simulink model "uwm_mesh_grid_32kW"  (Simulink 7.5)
settings: Solver=ode45  StartTime=0.0  StopTime=6.0  RelTol=1e-4
undefined symbols (not defined in the file or in its folder): bits, D1, Delta
libraries: powerlib x76, powerlib_extras x11, dspswit3 x4
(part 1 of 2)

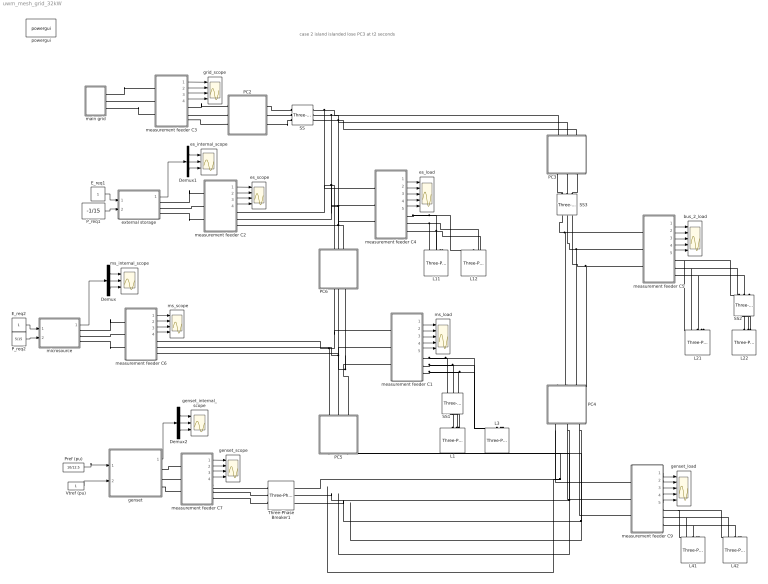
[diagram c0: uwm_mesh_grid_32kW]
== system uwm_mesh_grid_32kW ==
  note: case 2 island islanded lose PC3 at t2 seconds
  " es_scope" : Scope  NumInputPorts=4
  " ms_scope" : Scope  NumInputPorts=4
  Demux : Demux  Outputs=3
  Demux1 : Demux  Outputs=3
  Demux2 : Demux  Outputs=3
  E_req1 : Constant  OutDataType=fixdt(1, 16)  OutScaling=2^0
  E_req2 : Constant  OutDataType=fixdt(1, 16)  OutScaling=2^0
  L{1,3,11..12,21..22,41..42} (8 alike) : powerlib/Elements/Three-Phase Series RLC Load  DialogController=POWERSYS.PowerSysDialog  PhysicalDomain=powersysdomain  SubClassName=unknown  LeftPortType=p1  RightPortType=p1  LConnTagsString=A|B|C  Configuration=Y (grounded)  NominalVoltage=208  NominalFrequency=60  ActivePower=4000  InductivePower=0  CapacitivePower=0  Measurements=None
  PC2 : Subsystem  mask{R=.002810, L=.000679, C=2894.3}
  PC3 : Subsystem  mask{R=0.027352, L=.006600, C=288.6}
  PC4 : Subsystem  mask{R=.01688, L=.004070, C=336.7}
  PC5 : Subsystem  mask{R=.002600, L=.000640, C=2020.1}
  PC6 : Subsystem  mask{R=.013700, L=.003300, C=577.2}
  P_req1 : Constant  Value=-1/15  OutDataType=fixdt(1, 16)  OutScaling=2^0
  P_req2 : Constant  Value=5/15  OutDataType=fixdt(1, 16)  OutScaling=2^0
  Pref (pu) : Constant  Value=10/12.5  OutDataType=sfix(16)  OutScaling=2^0
  SS : powerlib/Elements/Three-Phase Breaker  DialogController=POWERSYS.PowerSysDialog  SystemSampleTime=-1  InitialState=closed  SwitchA=on  SwitchB=on  SwitchC=on  SwitchTimes=[3]  External=off  BreakerResistance=.001  SnubberResistance=1e6  SnubberCapacitance=inf  Measurements=None
  SS1 : powerlib/Elements/Three-Phase Breaker  DialogController=POWERSYS.PowerSysDialog  SystemSampleTime=-1  InitialState=closed  SwitchA=on  SwitchB=on  SwitchC=on  SwitchTimes=[50]  External=off  BreakerResistance=.001  SnubberResistance=1e6  SnubberCapacitance=inf  Measurements=None
  SS2 : powerlib/Elements/Three-Phase Breaker  DialogController=POWERSYS.PowerSysDialog  SystemSampleTime=-1  InitialState=closed  SwitchA=on  SwitchB=on  SwitchC=on  SwitchTimes=[50]  External=off  BreakerResistance=.00001  SnubberResistance=1e10  SnubberCapacitance=inf  Measurements=None
  SS3 : powerlib/Elements/Three-Phase Breaker  DialogController=POWERSYS.PowerSysDialog  SystemSampleTime=-1  InitialState=closed  SwitchA=on  SwitchB=on  SwitchC=on  SwitchTimes=[50]  External=off  BreakerResistance=.00001  SnubberResistance=1e10  SnubberCapacitance=inf  Measurements=None
  Three-Phase Breaker1 : powerlib/Elements/Three-Phase Breaker  DialogController=POWERSYS.PowerSysDialog  SystemSampleTime=-1  InitialState=closed  SwitchA=on  SwitchB=on  SwitchC=on  SwitchTimes=[50]  External=off  BreakerResistance=0.001  SnubberResistance=1e6  SnubberCapacitance=inf  Measurements=None
  Vtref (pu) : Constant  OutDataType=sfix(16)  OutScaling=2^0
  bus_2_load : Scope  NumInputPorts=5
  es_internal_scope : Scope  NumInputPorts=3
  es_load : Scope  NumInputPorts=5
  external storage : Subsystem  AncestorBlock=|
      | UWM_blocks/inverter-based
      | DG (simplified)
      | 208V - 15kVA
  genset : Subsystem
  genset_internal_scope : Scope  NumInputPorts=3
  genset_load : Scope  NumInputPorts=5
  genset_scope : Scope  NumInputPorts=4
  grid_scope : Scope  NumInputPorts=4
  main grid : Subsystem
  measurement feeder C1 : Subsystem
  measurement feeder C2 : Subsystem
  measurement feeder C3 : Subsystem
  measurement feeder C4 : Subsystem
  measurement feeder C5 : Subsystem
  measurement feeder C6 : Subsystem
  measurement feeder C7 : Subsystem
  measurement feeder C9 : Subsystem
  microsource : Subsystem  AncestorBlock=|
      | UWM_blocks/inverter-based
      | DG (simplified)
      | 208V - 15kVA
  ms_internal_scope : Scope  NumInputPorts=3
  ms_load : Scope  NumInputPorts=5
  powergui : powerlib/powergui  Priority=1  SystemSampleTime=-1  SimulationMode=Discrete  SampleTime=50e-6  frequency=60  SPID=off  DisableSnubberDevices=off  DisableRonSwitches=off  DisableVfSwitches=off  SwTol=0  Interpol=off  frequencyindice=60  echomessages=off  HookPort=off  DisplayEquations=off  FunctionMessages=off  EnableUseOfTLC=off  x0status=steady  RestoreLinks=no  ResistiveCurrentMeasurement=off  Frange=[0:2:500]  Ylog=off  Xlog=on  ShowGrid=off  save=off  variable=ZData  ZoomFFT=on  StartTime=0.0  cycles=1  DisplayStyle=1  fundamental=60  FreqAxis=off  MaxFrequency=1000  frequencyindicesteady=1  RmsSteady=2  display=off  Ts=0  methode=off
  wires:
  measurement feeder C3/1(Vabc) -> grid_scope/1
  measurement feeder C3/2(Iabc) -> grid_scope/2
  measurement feeder C3/3(PQ) -> grid_scope/3
  measurement feeder C3/4(RMS (V-I)) -> grid_scope/4
  measurement feeder C6/1(Vabc) -> " ms_scope"/1
  measurement feeder C6/2(Iabc) -> " ms_scope"/2
  measurement feeder C6/3(PQ) -> " ms_scope"/3
  measurement feeder C6/4(RMS (V-I)) -> " ms_scope"/4
  P_req2/1 -> microsource/2(P_req)
  E_req2/1 -> microsource/1(E_req)
  Demux/2 -> ms_internal_scope/2
  Demux/1 -> ms_internal_scope/1
  Demux/3 -> ms_internal_scope/3
  microsource/1(m) -> Demux/1
  P_req1/1 -> external storage/2(P_req)
  E_req1/1 -> external storage/1(E_req)
  Demux1/2 -> es_internal_scope/2
  Demux1/1 -> es_internal_scope/1
  Demux1/3 -> es_internal_scope/3
  external storage/1(m) -> Demux1/1
  measurement feeder C2/1(Vabc) -> " es_scope"/1
  measurement feeder C2/2(Iabc) -> " es_scope"/2
  measurement feeder C2/3(PQ) -> " es_scope"/3
  measurement feeder C2/4(RMS (V-I)) -> " es_scope"/4
  measurement feeder C4/5(w) -> es_load/5
  measurement feeder C4/4(RMS (V-I)) -> es_load/4
  measurement feeder C4/3(PQ) -> es_load/3
  measurement feeder C4/2(Iabc) -> es_load/2
  measurement feeder C4/1(Vabc) -> es_load/1
  measurement feeder C1/5(w) -> ms_load/5
  measurement feeder C1/4(RMS (V-I)) -> ms_load/4
  measurement feeder C1/3(PQ) -> ms_load/3
  measurement feeder C1/2(Iabc) -> ms_load/2
  measurement feeder C1/1(Vabc) -> ms_load/1
  measurement feeder C5/5(w) -> bus_2_load/5
  measurement feeder C5/4(RMS (V-I)) -> bus_2_load/4
  measurement feeder C5/3(PQ) -> bus_2_load/3
  measurement feeder C5/2(Iabc) -> bus_2_load/2
  measurement feeder C5/1(Vabc) -> bus_2_load/1
  measurement feeder C7/1(Vabc) -> genset_scope/1
  measurement feeder C7/2(Iabc) -> genset_scope/2
  measurement feeder C7/3(PQ) -> genset_scope/3
  measurement feeder C7/4(RMS (V-I)) -> genset_scope/4
  measurement feeder C9/5(w) -> genset_load/5
  measurement feeder C9/4(RMS (V-I)) -> genset_load/4
  measurement feeder C9/3(PQ) -> genset_load/3
  measurement feeder C9/1(Vabc) -> genset_load/1
  measurement feeder C9/2(Iabc) -> genset_load/2
  Vtref (pu)/1 -> genset/2(Ereq)
  Pref (pu)/1 -> genset/1(Preq)
  Demux2/2 -> genset_internal_scope/2
  Demux2/1 -> genset_internal_scope/1
  Demux2/3 -> genset_internal_scope/3
  genset/1(m) -> Demux2/1
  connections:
  SS/RConn3 -- measurement feeder C4/LConn3 -- measurement feeder C2/RConn3 -- PC6/RConn3 -- PC3/RConn3
  SS/RConn2 -- measurement feeder C4/LConn2 -- measurement feeder C2/RConn2 -- PC6/RConn2 -- PC3/RConn2
  SS/RConn1 -- measurement feeder C4/LConn1 -- measurement feeder C2/RConn1 -- PC6/RConn1 -- PC3/RConn1
  measurement feeder C4/RConn1 -- L12/LConn1 -- L11/LConn1
  measurement feeder C4/RConn2 -- L12/LConn2 -- L11/LConn2
  measurement feeder C4/RConn3 -- L12/LConn3 -- L11/LConn3
  measurement feeder C1/RConn1 -- L3/LConn1 -- SS1/LConn1
  measurement feeder C1/RConn2 -- L3/LConn2 -- SS1/LConn2
  measurement feeder C1/RConn3 -- L3/LConn3 -- SS1/LConn3
  measurement feeder C5/RConn1 -- SS2/LConn1 -- L21/LConn1
  measurement feeder C5/RConn2 -- SS2/LConn2 -- L21/LConn2
  measurement feeder C5/RConn3 -- SS2/LConn3 -- L21/LConn3
  measurement feeder C5/LConn1 -- PC4/RConn1 -- SS3/RConn1
  measurement feeder C5/LConn2 -- PC4/RConn2 -- SS3/RConn2
  measurement feeder C5/LConn3 -- PC4/RConn3 -- SS3/RConn3
  PC4/LConn1 -- measurement feeder C9/LConn1 -- Three-Phase Breaker1/RConn1 -- PC5/LConn1
  PC4/LConn2 -- measurement feeder C9/LConn2 -- Three-Phase Breaker1/RConn2 -- PC5/LConn2
  PC4/LConn3 -- measurement feeder C9/LConn3 -- Three-Phase Breaker1/RConn3 -- PC5/LConn3
  measurement feeder C9/RConn1 -- L41/LConn1 -- L42/LConn1
  measurement feeder C9/RConn2 -- L41/LConn2 -- L42/LConn2
  measurement feeder C9/RConn3 -- L41/LConn3 -- L42/LConn3
  PC5/RConn1 -- measurement feeder C6/RConn1 -- measurement feeder C1/LConn1 -- PC6/LConn1
  PC5/RConn2 -- measurement feeder C6/RConn2 -- measurement feeder C1/LConn2 -- PC6/LConn2
  microsource/RConn1 -- measurement feeder C6/LConn1
  PC5/RConn3 -- measurement feeder C6/RConn3 -- PC6/LConn3 -- measurement feeder C1/LConn3
  microsource/RConn2 -- measurement feeder C6/LConn2
  microsource/RConn3 -- measurement feeder C6/LConn3
  main grid/RConn2 -- measurement feeder C3/LConn2
  main grid/RConn1 -- measurement feeder C3/LConn1
  measurement feeder C3/LConn3 -- main grid/RConn3
  external storage/RConn2 -- measurement feeder C2/LConn2
  external storage/RConn1 -- measurement feeder C2/LConn1
  external storage/RConn3 -- measurement feeder C2/LConn3
  L1/LConn2 -- SS1/RConn2
  L1/LConn3 -- SS1/RConn3
  L1/LConn1 -- SS1/RConn1
  L22/LConn2 -- SS2/RConn2
  L22/LConn3 -- SS2/RConn3
  L22/LConn1 -- SS2/RConn1
  genset/RConn3 -- measurement feeder C7/LConn3
  genset/RConn1 -- measurement feeder C7/LConn1
  genset/RConn2 -- measurement feeder C7/LConn2
  measurement feeder C7/RConn1 -- Three-Phase Breaker1/LConn1
  Three-Phase Breaker1/LConn2 -- measurement feeder C7/RConn2
  Three-Phase Breaker1/LConn3 -- measurement feeder C7/RConn3
  measurement feeder C3/RConn1 -- PC2/LConn1
  measurement feeder C3/RConn2 -- PC2/LConn2
  measurement feeder C3/RConn3 -- PC2/LConn3
  PC2/RConn2 -- SS/LConn2
  PC2/RConn1 -- SS/LConn1
  SS/LConn3 -- PC2/RConn3
  SS3/LConn2 -- PC3/LConn2
  SS3/LConn3 -- PC3/LConn3
  SS3/LConn1 -- PC3/LConn1

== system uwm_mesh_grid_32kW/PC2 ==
  Ground : powerlib/Elements/Ground  DialogController=POWERSYS.PowerSysDialog  PhysicalDomain=powersysdomain  SubClassName=unknown  LeftPortType=p1  RightPortType=p1  LConnTagsString=a
  Three-Phase Parallel RLC Branch : powerlib/Elements/Three-Phase Parallel RLC Branch  DialogController=POWERSYS.PowerSysDialog  PhysicalDomain=powersysdomain  SubClassName=unknown  LeftPortType=p1  RightPortType=p1  LConnTagsString=A|B|C  RConnTagsString=A|B|C  BranchType=C  Resistance=1  Inductance=1e-3  Capacitance=1/(C*2*pi*60)  Measurements=None
  Three-Phase Series RLC Branch3 : powerlib/Elements/Three-Phase Series RLC Branch  DialogController=POWERSYS.PowerSysDialog  PhysicalDomain=powersysdomain  SubClassName=unknown  LeftPortType=p1  RightPortType=p1  LConnTagsString=A|B|C  RConnTagsString=A|B|C  BranchType=RL  Resistance=R  Inductance=L/(2*pi*60)  Capacitance=1/(336*2*pi*60)  Measurements=None
  A* : PMIOPort  Tag=PMCPort  Port=1  Side=Right
  B* : PMIOPort  Tag=PMCPort  Port=2  Side=Right
  C* : PMIOPort  Tag=PMCPort  Port=3  Side=Right
  A : PMIOPort  Tag=PMCPort  Port=4  Side=Left
  B : PMIOPort  Tag=PMCPort  Port=5  Side=Left
  C : PMIOPort  Tag=PMCPort  Port=6  Side=Left
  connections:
  Three-Phase Parallel RLC Branch/LConn1 -- A*/RConn1 -- Three-Phase Series RLC Branch3/LConn1
  Three-Phase Parallel RLC Branch/LConn2 -- B*/RConn1 -- Three-Phase Series RLC Branch3/LConn2
  Three-Phase Parallel RLC Branch/LConn3 -- C*/RConn1 -- Three-Phase Series RLC Branch3/LConn3
  Three-Phase Series RLC Branch3/RConn1 -- A/RConn1
  Three-Phase Series RLC Branch3/RConn2 -- B/RConn1
  Three-Phase Series RLC Branch3/RConn3 -- C/RConn1
  Ground/LConn1 -- Three-Phase Parallel RLC Branch/RConn2 -- Three-Phase Parallel RLC Branch/RConn3 -- Three-Phase Parallel RLC Branch/RConn1

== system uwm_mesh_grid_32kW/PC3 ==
  Ground : powerlib/Elements/Ground  DialogController=POWERSYS.PowerSysDialog  PhysicalDomain=powersysdomain  SubClassName=unknown  LeftPortType=p1  RightPortType=p1  LConnTagsString=a
  Three-Phase Parallel RLC Branch : powerlib/Elements/Three-Phase Parallel RLC Branch  DialogController=POWERSYS.PowerSysDialog  PhysicalDomain=powersysdomain  SubClassName=unknown  LeftPortType=p1  RightPortType=p1  LConnTagsString=A|B|C  RConnTagsString=A|B|C  BranchType=C  Resistance=1  Inductance=1e-3  Capacitance=1/(C*2*pi*60)  Measurements=None
  Three-Phase Series RLC Branch3 : powerlib/Elements/Three-Phase Series RLC Branch  DialogController=POWERSYS.PowerSysDialog  PhysicalDomain=powersysdomain  SubClassName=unknown  LeftPortType=p1  RightPortType=p1  LConnTagsString=A|B|C  RConnTagsString=A|B|C  BranchType=RL  Resistance=R  Inductance=L/(2*pi*60)  Capacitance=1/(336*2*pi*60)  Measurements=None
  A* : PMIOPort  Tag=PMCPort  Port=1  Side=Right
  B* : PMIOPort  Tag=PMCPort  Port=2  Side=Right
  C* : PMIOPort  Tag=PMCPort  Port=3  Side=Right
  A : PMIOPort  Tag=PMCPort  Port=4  Side=Left
  B : PMIOPort  Tag=PMCPort  Port=5  Side=Left
  C : PMIOPort  Tag=PMCPort  Port=6  Side=Left
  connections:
  Three-Phase Parallel RLC Branch/LConn1 -- A*/RConn1 -- Three-Phase Series RLC Branch3/LConn1
  Three-Phase Parallel RLC Branch/LConn2 -- B*/RConn1 -- Three-Phase Series RLC Branch3/LConn2
  Three-Phase Parallel RLC Branch/LConn3 -- C*/RConn1 -- Three-Phase Series RLC Branch3/LConn3
  Three-Phase Series RLC Branch3/RConn1 -- A/RConn1
  Three-Phase Series RLC Branch3/RConn2 -- B/RConn1
  Three-Phase Series RLC Branch3/RConn3 -- C/RConn1
  Ground/LConn1 -- Three-Phase Parallel RLC Branch/RConn2 -- Three-Phase Parallel RLC Branch/RConn1 -- Three-Phase Parallel RLC Branch/RConn3

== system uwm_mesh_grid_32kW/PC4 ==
  Ground : powerlib/Elements/Ground  DialogController=POWERSYS.PowerSysDialog  PhysicalDomain=powersysdomain  SubClassName=unknown  LeftPortType=p1  RightPortType=p1  LConnTagsString=a
  Three-Phase Parallel RLC Branch : powerlib/Elements/Three-Phase Parallel RLC Branch  DialogController=POWERSYS.PowerSysDialog  PhysicalDomain=powersysdomain  SubClassName=unknown  LeftPortType=p1  RightPortType=p1  LConnTagsString=A|B|C  RConnTagsString=A|B|C  BranchType=C  Resistance=1  Inductance=1e-3  Capacitance=1/(C*2*pi*60)  Measurements=None
  Three-Phase Series RLC Branch3 : powerlib/Elements/Three-Phase Series RLC Branch  DialogController=POWERSYS.PowerSysDialog  PhysicalDomain=powersysdomain  SubClassName=unknown  LeftPortType=p1  RightPortType=p1  LConnTagsString=A|B|C  RConnTagsString=A|B|C  BranchType=RL  Resistance=R  Inductance=L/(2*pi*60)  Capacitance=1/(336*2*pi*60)  Measurements=None
  A* : PMIOPort  Tag=PMCPort  Port=1  Side=Right
  B* : PMIOPort  Tag=PMCPort  Port=2  Side=Right
  C* : PMIOPort  Tag=PMCPort  Port=3  Side=Right
  A : PMIOPort  Tag=PMCPort  Port=4  Side=Left
  B : PMIOPort  Tag=PMCPort  Port=5  Side=Left
  C : PMIOPort  Tag=PMCPort  Port=6  Side=Left
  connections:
  A*/RConn1 -- Three-Phase Series RLC Branch3/LConn1 -- Three-Phase Parallel RLC Branch/LConn1
  B*/RConn1 -- Three-Phase Series RLC Branch3/LConn2 -- Three-Phase Parallel RLC Branch/LConn2
  C*/RConn1 -- Three-Phase Series RLC Branch3/LConn3 -- Three-Phase Parallel RLC Branch/LConn3
  Three-Phase Series RLC Branch3/RConn1 -- A/RConn1
  Three-Phase Series RLC Branch3/RConn2 -- B/RConn1
  Three-Phase Series RLC Branch3/RConn3 -- C/RConn1
  Ground/LConn1 -- Three-Phase Parallel RLC Branch/RConn2 -- Three-Phase Parallel RLC Branch/RConn3 -- Three-Phase Parallel RLC Branch/RConn1

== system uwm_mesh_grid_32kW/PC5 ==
  Ground : powerlib/Elements/Ground  DialogController=POWERSYS.PowerSysDialog  PhysicalDomain=powersysdomain  SubClassName=unknown  LeftPortType=p1  RightPortType=p1  LConnTagsString=a
  Three-Phase Parallel RLC Branch : powerlib/Elements/Three-Phase Parallel RLC Branch  DialogController=POWERSYS.PowerSysDialog  PhysicalDomain=powersysdomain  SubClassName=unknown  LeftPortType=p1  RightPortType=p1  LConnTagsString=A|B|C  RConnTagsString=A|B|C  BranchType=C  Resistance=1  Inductance=1e-3  Capacitance=1/(C*2*pi*60)  Measurements=None
  Three-Phase Series RLC Branch3 : powerlib/Elements/Three-Phase Series RLC Branch  DialogController=POWERSYS.PowerSysDialog  PhysicalDomain=powersysdomain  SubClassName=unknown  LeftPortType=p1  RightPortType=p1  LConnTagsString=A|B|C  RConnTagsString=A|B|C  BranchType=RL  Resistance=R  Inductance=L/(2*pi*60)  Capacitance=1/(336*2*pi*60)  Measurements=None
  A* : PMIOPort  Tag=PMCPort  Port=1  Side=Right
  B* : PMIOPort  Tag=PMCPort  Port=2  Side=Right
  C* : PMIOPort  Tag=PMCPort  Port=3  Side=Right
  A : PMIOPort  Tag=PMCPort  Port=4  Side=Left
  B : PMIOPort  Tag=PMCPort  Port=5  Side=Left
  C : PMIOPort  Tag=PMCPort  Port=6  Side=Left
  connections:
  Three-Phase Parallel RLC Branch/LConn1 -- A*/RConn1 -- Three-Phase Series RLC Branch3/LConn1
  Three-Phase Parallel RLC Branch/LConn2 -- B*/RConn1 -- Three-Phase Series RLC Branch3/LConn2
  Three-Phase Parallel RLC Branch/LConn3 -- C*/RConn1 -- Three-Phase Series RLC Branch3/LConn3
  Three-Phase Series RLC Branch3/RConn1 -- A/RConn1
  Three-Phase Series RLC Branch3/RConn2 -- B/RConn1
  Three-Phase Series RLC Branch3/RConn3 -- C/RConn1
  Ground/LConn1 -- Three-Phase Parallel RLC Branch/RConn2 -- Three-Phase Parallel RLC Branch/RConn3 -- Three-Phase Parallel RLC Branch/RConn1

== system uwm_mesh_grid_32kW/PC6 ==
  Ground : powerlib/Elements/Ground  DialogController=POWERSYS.PowerSysDialog  PhysicalDomain=powersysdomain  SubClassName=unknown  LeftPortType=p1  RightPortType=p1  LConnTagsString=a
  Three-Phase Parallel RLC Branch : powerlib/Elements/Three-Phase Parallel RLC Branch  DialogController=POWERSYS.PowerSysDialog  PhysicalDomain=powersysdomain  SubClassName=unknown  LeftPortType=p1  RightPortType=p1  LConnTagsString=A|B|C  RConnTagsString=A|B|C  BranchType=C  Resistance=1  Inductance=1e-3  Capacitance=1/(C*2*pi*60)  Measurements=None
  Three-Phase Series RLC Branch3 : powerlib/Elements/Three-Phase Series RLC Branch  DialogController=POWERSYS.PowerSysDialog  PhysicalDomain=powersysdomain  SubClassName=unknown  LeftPortType=p1  RightPortType=p1  LConnTagsString=A|B|C  RConnTagsString=A|B|C  BranchType=RL  Resistance=R  Inductance=L/(2*pi*60)  Capacitance=1/(336*2*pi*60)  Measurements=None
  A* : PMIOPort  Tag=PMCPort  Port=1  Side=Right
  B* : PMIOPort  Tag=PMCPort  Port=2  Side=Right
  C* : PMIOPort  Tag=PMCPort  Port=3  Side=Right
  A : PMIOPort  Tag=PMCPort  Port=4  Side=Left
  B : PMIOPort  Tag=PMCPort  Port=5  Side=Left
  C : PMIOPort  Tag=PMCPort  Port=6  Side=Left
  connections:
  Three-Phase Parallel RLC Branch/LConn1 -- A*/RConn1 -- Three-Phase Series RLC Branch3/LConn1
  Three-Phase Parallel RLC Branch/LConn2 -- B*/RConn1 -- Three-Phase Series RLC Branch3/LConn2
  Three-Phase Parallel RLC Branch/LConn3 -- C*/RConn1 -- Three-Phase Series RLC Branch3/LConn3
  Three-Phase Series RLC Branch3/RConn1 -- A/RConn1
  Three-Phase Series RLC Branch3/RConn2 -- B/RConn1
  Three-Phase Series RLC Branch3/RConn3 -- C/RConn1
  Ground/LConn1 -- Three-Phase Parallel RLC Branch/RConn2 -- Three-Phase Parallel RLC Branch/RConn3 -- Three-Phase Parallel RLC Branch/RConn1

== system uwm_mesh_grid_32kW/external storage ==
  E_req : Inport
  P_req : Inport  Port=2
  10 mH : powerlib/Elements/Three-Phase Series RLC Branch  DialogController=POWERSYS.PowerSysDialog  PhysicalDomain=powersysdomain  SubClassName=unknown  LeftPortType=p1  RightPortType=p1  LConnTagsString=A|B|C  RConnTagsString=A|B|C  BranchType=L  Resistance=.0028  Inductance=5e-3  Capacitance=1e-6  Measurements=None
  Current Measurement : powerlib/Measurements/Current Measurement  DialogController=POWERSYS.PowerSysDialog  SystemSampleTime=-1  PhasorSimulation=off  OutputType=Complex  PSBequivalent=0
  Gain : Gain  Gain=1/(2*pi)  ParameterDataType=fixdt(1, 16)  ParameterScaling=2^0  OutDataType=fixdt(1, 16)  OutScaling=2^0
  Mux : Mux  Inputs=3
  T1 : powerlib/Elements/Three-Phase Transformer (Two Windings)  DialogController=POWERSYS.PowerSysDialog  SystemSampleTime=-1  Winding1Connection=Delta (D1)  UNITS=SI  NominalPower=[ 45e3 , 60 ]  Winding1=[208 0.02688 0.1075/(2*pi*60)]  Winding2Connection=Yg  Winding2=[208 0.005047 .0201/(2*pi*60)]  SetSaturation=off  Rm=100.e6  Lm=7650.8  Saturation=[0 0;1359.8 0.93633;5.6659e+05 1.186]  Hysteresis=off  DataFile='hysteresis'  SetInitialFlux=off  InitialFluxes=[0.62422 -0.62422 0.54618]  Measurements=None  MoreParameters=off  BreakLoop=off  DataType=on  TransfoNumber=1
  Three-Phase V-I Measurement : powerlib/Measurements/Three-Phase V-I Measurement  DialogController=POWERSYS.PowerSysDialog  SystemSampleTime=-1  VoltageMeasurement=phase-to-ground  SetLabelV=off  LabelV=Vabc  Vpu=off  VpuLL=off  CurrentMeasurement=yes  SetLabelI=off  LabelI=Iabc  Ipu=off  Pbase=100e6  Vbase=500e3  OutputType=Complex  PhasorSimulation=off  PSBequivalent=0
  UWM_controller : Subsystem  mask{Vbase=208, Sbase=15000}
  Voltage Measurement : powerlib/Measurements/Voltage Measurement  DialogController=POWERSYS.PowerSysDialog  SystemSampleTime=-1  PhasorSimulation=off  OutputType=Complex  PSBequivalent=0
  microsource : Subsystem
  a : PMIOPort  Port=1  Side=Right
  b : PMIOPort  Port=2  Side=Right
  c : PMIOPort  Port=3  Side=Right
  m : Outport  OutDataType=fixdt(1, 16)  OutScaling=2^0
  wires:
  E_req/1 -> UWM_controller/3(E_req)
  P_req/1 -> UWM_controller/4(P_req)
  Three-Phase V-I Measurement/1 -> UWM_controller/1(v_meas)
  Three-Phase V-I Measurement/2 -> UWM_controller/2(i_meas)
  UWM_controller/1(Vpk) -> microsource/1(Vpk)
  UWM_controller/2(w) -> microsource/2(w), Gain/1
  Mux/1 -> m/1
  Voltage Measurement/1 -> Mux/1
  Current Measurement/1 -> Mux/2
  Gain/1 -> Mux/3
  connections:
  Three-Phase V-I Measurement/RConn2 -- b/RConn1 -- Voltage Measurement/LConn2
  Three-Phase V-I Measurement/RConn3 -- c/RConn1
  Current Measurement/RConn1 -- a/RConn1
  Three-Phase V-I Measurement/RConn1 -- Current Measurement/LConn1 -- Voltage Measurement/LConn1
  10 mH/LConn2 -- microsource/RConn2
  10 mH/LConn1 -- microsource/RConn1
  10 mH/LConn3 -- microsource/RConn3
  T1/LConn1 -- 10 mH/RConn1
  T1/LConn2 -- 10 mH/RConn2
  T1/LConn3 -- 10 mH/RConn3
  T1/RConn1 -- Three-Phase V-I Measurement/LConn1
  T1/RConn2 -- Three-Phase V-I Measurement/LConn2
  T1/RConn3 -- Three-Phase V-I Measurement/LConn3

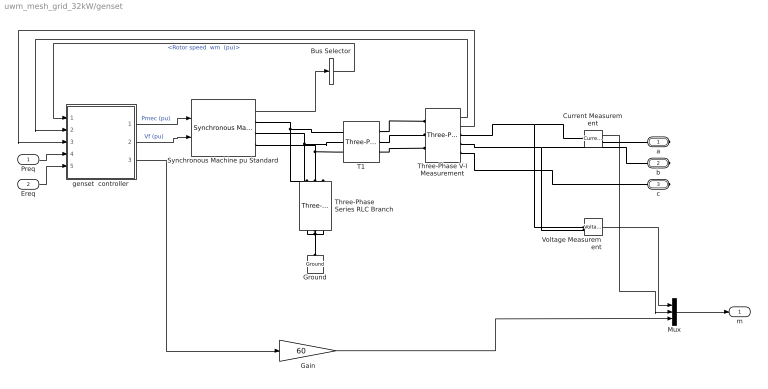
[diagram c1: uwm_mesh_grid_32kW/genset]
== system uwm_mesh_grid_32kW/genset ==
  Preq : Inport  OutDataType=fixdt(1, 16)  OutScaling=2^0
  Ereq : Inport  Port=2  OutDataType=fixdt(1, 16)  OutScaling=2^0
  Bus Selector : BusSelector  OutputSignals="Mechanical.Rotor speed  wm  (pu)"
  Current Measurement : powerlib/Measurements/Current Measurement  DialogController=POWERSYS.PowerSysDialog  SystemSampleTime=-1  PhasorSimulation=off  OutputType=Complex  PSBequivalent=0
  Gain : Gain  Gain=60  ParameterDataType=fixdt(1, 16)  ParameterScaling=2^0  OutDataType=fixdt(1, 16)  OutScaling=2^0
  Ground : powerlib/Elements/Ground  DialogController=POWERSYS.PowerSysDialog  PhysicalDomain=powersysdomain  SubClassName=unknown  LeftPortType=p1  RightPortType=p1  LConnTagsString=a
  Mux : Mux  Inputs=3
  Synchronous Machine pu Standard : powerlib/Machines/Synchronous Machine pu Standard  DialogController=POWERSYS.PowerSysDialog  SystemSampleTime=-1  PresetModel=No  MechanicalLoad=Mechanical power Pm  ShowDetailedParameters=on  RotorType=Salient-pole  NominalParameters="[ 12500  208   60]"  Reactances1=[ 1.81, 0.3, 0.23, 1.76, 0.65, 0.25, 0.15 ]  Reactances2="[ 1.204, 0.125, 0.056, 0.533,  0.051,  0.037 ]"  dAxisTimeConstants=Short-circuit  qAxisTimeConstants=Short-circuit  TimeConstants1="[ 4.4849  0.0681  0.1  ]"  TimeConstants2=[ 8.0, 0.03, 1.0, 0.07 ]  TimeConstants3="[  .35523  0.00015  0.067  ]"  TimeConstants4=[ 8.0, 0.03, 0.3371, 0.0295 ]  TimeConstants5=[ 1.01, 0.053, 0.1 ]  TimeConstants6=[ 1.3201, 0.023, 1.0, 0.07 ]  TimeConstants7=[0.35523 0.00015 0.0067]  TimeConstants8=[ 1.3201, 0.0231, 0.3371, 0.0295 ]  StatorResistance=0.0217  Mechanical=[ .19 0 2 ]  PolePairs=2  InitialConditions="[ 0  0  0  0  0  0  0  0  1 ]"  SetSaturation=off  Saturation=[0.6404,0.7127,0.8441,0.9214,0.9956,1.082,1.19,1.316,1.457;0.7,0.7698,0.8872,0.9466,0.9969,1.046,1.1,1.151,1.201]  Units=per unit standard parameters  LoadFlowParameters=[1 0 0 0 0]  TsPowergui=0  TsBlock=-1  IterativeModel=Forward Euler
  T1 : powerlib/Elements/Three-Phase Transformer (Two Windings)  DialogController=POWERSYS.PowerSysDialog  SystemSampleTime=-1  Winding1Connection=Delta (D1)  UNITS=SI  NominalPower=[ 45e3 , 60 ]  Winding1=[208 .02688 .10752/(2*pi*60)]  Winding2Connection=Yg  Winding2=[208 .005047 .201899/(2*pi*60)]  SetSaturation=off  Rm=1e+08  Lm=7650.8  Saturation=[0 0;1359.8 0.93633;5.6659e+05 1.186]  Hysteresis=off  DataFile='hysteresis'  SetInitialFlux=off  InitialFluxes=[0.62422 -0.62422 0.54618]  Measurements=None  MoreParameters=off  BreakLoop=off  DataType=on  TransfoNumber=1
  Three-Phase Series RLC Branch : powerlib/Elements/Three-Phase Series RLC Branch  DialogController=POWERSYS.PowerSysDialog  PhysicalDomain=powersysdomain  SubClassName=unknown  LeftPortType=p1  RightPortType=p1  LConnTagsString=A|B|C  RConnTagsString=A|B|C  BranchType=C  Resistance=1  Inductance=1e-3  Capacitance=1.e-4  Measurements=None
  Three-Phase V-I Measurement : powerlib/Measurements/Three-Phase V-I Measurement  DialogController=POWERSYS.PowerSysDialog  SystemSampleTime=-1  VoltageMeasurement=phase-to-ground  SetLabelV=off  LabelV=Vabc  Vpu=off  VpuLL=off  CurrentMeasurement=yes  SetLabelI=off  LabelI=Iabc  Ipu=off  Pbase=100e6  Vbase=500e3  OutputType=Complex  PhasorSimulation=off  PSBequivalent=0
  Voltage Measurement : powerlib/Measurements/Voltage Measurement  DialogController=POWERSYS.PowerSysDialog  SystemSampleTime=-1  PhasorSimulation=off  OutputType=Complex  PSBequivalent=0
  genset  controller : Subsystem  mask{Vbase=208, Sbase=12500}
  a : PMIOPort  Port=1  Side=Right
  b : PMIOPort  Port=2  Side=Right
  c : PMIOPort  Port=3  Side=Right
  m : Outport  OutDataType=fixdt(1, 16)  OutScaling=2^0
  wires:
  genset  controller/1(Pmech) -> Synchronous Machine pu Standard/1  "Pmec (pu)"
  genset  controller/2(Vf) -> Synchronous Machine pu Standard/2  "Vf (pu)"
  Synchronous Machine pu Standard/1 -> Bus Selector/1
  Bus Selector/1 -> genset  controller/1(wr)  "<Rotor speed  wm  (pu)>"
  Three-Phase V-I Measurement/1 -> genset  controller/2(Vabc)
  Three-Phase V-I Measurement/2 -> genset  controller/3(Iabc)
  Preq/1 -> genset  controller/4(Preq)
  Ereq/1 -> genset  controller/5(Ereq1)
  Mux/1 -> m/1
  Voltage Measurement/1 -> Mux/1
  Current Measurement/1 -> Mux/2
  genset  controller/3(w) -> Gain/1
  Gain/1 -> Mux/3
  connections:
  Three-Phase V-I Measurement/RConn1 -- Current Measurement/LConn1 -- Voltage Measurement/LConn1
  Three-Phase V-I Measurement/RConn2 -- b/RConn1 -- Voltage Measurement/LConn2
  Three-Phase V-I Measurement/RConn3 -- c/RConn1
  Three-Phase Series RLC Branch/RConn2 -- Three-Phase Series RLC Branch/RConn1 -- Ground/LConn1 -- Three-Phase Series RLC Branch/RConn3
  Synchronous Machine pu Standard/RConn1 -- T1/LConn1 -- Three-Phase Series RLC Branch/LConn1
  Synchronous Machine pu Standard/RConn2 -- T1/LConn2 -- Three-Phase Series RLC Branch/LConn2
  Synchronous Machine pu Standard/RConn3 -- T1/LConn3 -- Three-Phase Series RLC Branch/LConn3
  T1/RConn2 -- Three-Phase V-I Measurement/LConn2
  T1/RConn1 -- Three-Phase V-I Measurement/LConn1
  T1/RConn3 -- Three-Phase V-I Measurement/LConn3
  Current Measurement/RConn1 -- a/RConn1

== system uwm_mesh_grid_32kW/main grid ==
  4.16kV 2500kVA : powerlib/Electrical Sources/Three-Phase Source  DialogController=POWERSYS.PowerSysDialog  SystemSampleTime=-1  Voltage=4160  PhaseAngle=0  Frequency=60  InternalConnection=Yg  SpecifyImpedance=on  Resistance=25^2/1000/10  Inductance=25^2/1000/377  ShortCircuitLevel=1200e6  BaseVoltage=4160  XRratio=100
  PC1 : Subsystem  mask{R=.093400, L=.025500, C=2894.3}
  T1 : powerlib/Elements/Three-Phase Transformer (Two Windings)  DialogController=POWERSYS.PowerSysDialog  SystemSampleTime=-1  Winding1Connection=Delta (D1)  UNITS=SI  NominalPower=[ 2500e3 , 60 ]  Winding1=[4160 .04706 .1882/(2*pi*60)]  Winding2Connection=Yg  Winding2=[480 .000627 .0025068/(2*pi*60)]  SetSaturation=off  Rm=1.e6  Lm=1.e6  Saturation=[0 0;589.26 2.1608;2.4552e+05 2.737]  Hysteresis=off  DataFile='hysteresis'  SetInitialFlux=off  InitialFluxes=[1.4405 -1.4405 1.2604]  Measurements=None  MoreParameters=off  BreakLoop=off  DataType=on  TransfoNumber=1
  T2 : powerlib/Elements/Three-Phase Transformer (Two Windings)  DialogController=POWERSYS.PowerSysDialog  SystemSampleTime=-1  Winding1Connection=Delta (D1)  UNITS=SI  NominalPower=[ 75e3 , 60 ]  Winding1=[480 .0169 .0676/(2*pi*60)]  Winding2Connection=Yg  Winding2=[208 .0003 .0127/(2*pi*60)]  SetSaturation=off  Rm=1.e6  Lm=1.e6  Saturation=[0 0;589.26 2.1608;2.4552e+05 2.737]  Hysteresis=off  DataFile='hysteresis'  SetInitialFlux=off  InitialFluxes=[1.4405 -1.4405 1.2604]  Measurements=None  MoreParameters=off  BreakLoop=off  DataType=on  TransfoNumber=1
  A : PMIOPort  Port=1  Side=Right
  B : PMIOPort  Port=2  Side=Right
  C : PMIOPort  Port=3  Side=Right
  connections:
  A/RConn1 -- T2/RConn1
  B/RConn1 -- T2/RConn2
  C/RConn1 -- T2/RConn3
  T1/RConn1 -- PC1/LConn1
  T1/RConn2 -- PC1/LConn2
  T1/RConn3 -- PC1/LConn3
  PC1/RConn1 -- T2/LConn1
  PC1/RConn2 -- T2/LConn2
  PC1/RConn3 -- T2/LConn3
  4.16kV 2500kVA/RConn2 -- T1/LConn2
  4.16kV 2500kVA/RConn1 -- T1/LConn1
  4.16kV 2500kVA/RConn3 -- T1/LConn3

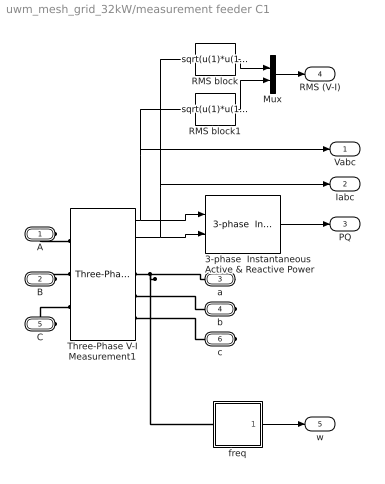
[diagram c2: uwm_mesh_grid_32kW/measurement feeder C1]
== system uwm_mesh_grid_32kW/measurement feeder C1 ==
  3-phase  Instantaneous  Active & Reactive Power : powerlib_extras/Measurements/3-phase  Instantaneous  Active & Reactive Power  DialogController=POWERSYS.PowerSysDialog  SystemSampleTime=-1
  Mux : Mux  Inputs=2
  RMS block : Fcn  Expr=sqrt(u(1)*u(1)+u(2)*u(2)+u(3)*u(3))/sqrt(3)
  RMS block1 : Fcn  Expr=sqrt(u(1)*u(1)+u(2)*u(2)+u(3)*u(3))/sqrt(3)
  Three-Phase V-I Measurement1 : powerlib/Measurements/Three-Phase V-I Measurement  DialogController=POWERSYS.PowerSysDialog  SystemSampleTime=-1  VoltageMeasurement=phase-to-ground  SetLabelV=off  LabelV=Vabc  Vpu=off  VpuLL=off  CurrentMeasurement=yes  SetLabelI=off  LabelI=Iabc  Ipu=off  Pbase=100e6  Vbase=500e3  OutputType=Complex  PhasorSimulation=off  PSBequivalent=0
  freq : Subsystem  AncestorBlock=|
      | UWM_blocks/frequency
      | measurement
      | (zero-crossings)
  A : PMIOPort  Port=1  Side=Left
  B : PMIOPort  Port=2  Side=Left
  a : PMIOPort  Port=3  Side=Right
  b : PMIOPort  Port=4  Side=Right
  C : PMIOPort  Port=5  Side=Left
  c : PMIOPort  Port=6  Side=Right
  Vabc : Outport  OutDataType=fixdt(1, 16)  OutScaling=2^0
  Iabc : Outport  Port=2  OutDataType=fixdt(1, 16)  OutScaling=2^0
  PQ : Outport  Port=3  OutDataType=fixdt(1, 16)  OutScaling=2^0
  RMS (V-I) : Outport  Port=4  OutDataType=fixdt(1, 16)  OutScaling=2^0
  w : Outport  Port=5  OutDataType=fixdt(1, 16)  OutScaling=2^0
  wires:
  Three-Phase V-I Measurement1/1 -> Vabc/1, RMS block1/1, 3-phase  Instantaneous  Active & Reactive Power/1
  Three-Phase V-I Measurement1/2 -> Iabc/1, RMS block/1, 3-phase  Instantaneous  Active & Reactive Power/2
  Mux/1 -> RMS (V-I)/1
  RMS block/1 -> Mux/1
  RMS block1/1 -> Mux/2
  3-phase  Instantaneous  Active & Reactive Power/1 -> PQ/1
  freq/1(w (Hz)) -> w/1
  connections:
  c/RConn1 -- Three-Phase V-I Measurement1/RConn3
  C/RConn1 -- Three-Phase V-I Measurement1/LConn3
  b/RConn1 -- Three-Phase V-I Measurement1/RConn2
  Three-Phase V-I Measurement1/RConn1 -- a/RConn1 -- freq/LConn1
  B/RConn1 -- Three-Phase V-I Measurement1/LConn2
  A/RConn1 -- Three-Phase V-I Measurement1/LConn1

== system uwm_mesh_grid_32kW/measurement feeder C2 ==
  3-phase  Instantaneous  Active & Reactive Power : powerlib_extras/Measurements/3-phase  Instantaneous  Active & Reactive Power  DialogController=POWERSYS.PowerSysDialog  SystemSampleTime=-1
  Mux : Mux  Inputs=2
  RMS block : Fcn  Expr=sqrt(u(1)*u(1)+u(2)*u(2)+u(3)*u(3))/sqrt(3)
  RMS block1 : Fcn  Expr=sqrt(u(1)*u(1)+u(2)*u(2)+u(3)*u(3))/sqrt(3)
  Three-Phase V-I Measurement : powerlib/Measurements/Three-Phase V-I Measurement  DialogController=POWERSYS.PowerSysDialog  SystemSampleTime=-1  VoltageMeasurement=phase-to-ground  SetLabelV=off  LabelV=Vabc  Vpu=off  VpuLL=off  CurrentMeasurement=yes  SetLabelI=off  LabelI=Iabc  Ipu=off  Pbase=100e6  Vbase=500e3  OutputType=Complex  PhasorSimulation=off  PSBequivalent=0
  A : PMIOPort  Port=1  Side=Left
  B : PMIOPort  Port=2  Side=Left
  a : PMIOPort  Port=3  Side=Right
  b : PMIOPort  Port=4  Side=Right
  C : PMIOPort  Port=5  Side=Left
  c : PMIOPort  Port=6  Side=Right
  Vabc : Outport  OutDataType=fixdt(1, 16)  OutScaling=2^0
  Iabc : Outport  Port=2  OutDataType=fixdt(1, 16)  OutScaling=2^0
  PQ : Outport  Port=3  OutDataType=fixdt(1, 16)  OutScaling=2^0
  RMS (V-I) : Outport  Port=4  OutDataType=fixdt(1, 16)  OutScaling=2^0
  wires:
  Three-Phase V-I Measurement/1 -> Vabc/1, RMS block1/1, 3-phase  Instantaneous  Active & Reactive Power/1
  Three-Phase V-I Measurement/2 -> Iabc/1, RMS block/1, 3-phase  Instantaneous  Active & Reactive Power/2
  Mux/1 -> RMS (V-I)/1
  RMS block/1 -> Mux/1
  RMS block1/1 -> Mux/2
  3-phase  Instantaneous  Active & Reactive Power/1 -> PQ/1
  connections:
  c/RConn1 -- Three-Phase V-I Measurement/RConn3
  C/RConn1 -- Three-Phase V-I Measurement/LConn3
  b/RConn1 -- Three-Phase V-I Measurement/RConn2
  a/RConn1 -- Three-Phase V-I Measurement/RConn1
  B/RConn1 -- Three-Phase V-I Measurement/LConn2
  A/RConn1 -- Three-Phase V-I Measurement/LConn1

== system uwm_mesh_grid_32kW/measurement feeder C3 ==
  3-phase  Instantaneous  Active & Reactive Power : powerlib_extras/Measurements/3-phase  Instantaneous  Active & Reactive Power  DialogController=POWERSYS.PowerSysDialog  SystemSampleTime=-1
  Mux : Mux  Inputs=2
  RMS block : Fcn  Expr=sqrt(u(1)*u(1)+u(2)*u(2)+u(3)*u(3))/sqrt(3)
  RMS block1 : Fcn  Expr=sqrt(u(1)*u(1)+u(2)*u(2)+u(3)*u(3))/sqrt(3)
  Three-Phase V-I Measurement : powerlib/Measurements/Three-Phase V-I Measurement  DialogController=POWERSYS.PowerSysDialog  SystemSampleTime=-1  VoltageMeasurement=phase-to-ground  SetLabelV=off  LabelV=Vabc  Vpu=off  VpuLL=off  CurrentMeasurement=yes  SetLabelI=off  LabelI=Iabc  Ipu=off  Pbase=100e6  Vbase=500e3  OutputType=Complex  PhasorSimulation=off  PSBequivalent=0
  A : PMIOPort  Port=1  Side=Left
  B : PMIOPort  Port=2  Side=Left
  a : PMIOPort  Port=3  Side=Right
  b : PMIOPort  Port=4  Side=Right
  C : PMIOPort  Port=5  Side=Left
  c : PMIOPort  Port=6  Side=Right
  Vabc : Outport  OutDataType=fixdt(1, 16)  OutScaling=2^0
  Iabc : Outport  Port=2  OutDataType=fixdt(1, 16)  OutScaling=2^0
  PQ : Outport  Port=3  OutDataType=fixdt(1, 16)  OutScaling=2^0
  RMS (V-I) : Outport  Port=4  OutDataType=fixdt(1, 16)  OutScaling=2^0
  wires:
  Three-Phase V-I Measurement/1 -> Vabc/1, RMS block1/1, 3-phase  Instantaneous  Active & Reactive Power/1
  Three-Phase V-I Measurement/2 -> Iabc/1, RMS block/1, 3-phase  Instantaneous  Active & Reactive Power/2
  Mux/1 -> RMS (V-I)/1
  RMS block/1 -> Mux/1
  RMS block1/1 -> Mux/2
  3-phase  Instantaneous  Active & Reactive Power/1 -> PQ/1
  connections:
  c/RConn1 -- Three-Phase V-I Measurement/RConn3
  C/RConn1 -- Three-Phase V-I Measurement/LConn3
  b/RConn1 -- Three-Phase V-I Measurement/RConn2
  a/RConn1 -- Three-Phase V-I Measurement/RConn1
  B/RConn1 -- Three-Phase V-I Measurement/LConn2
  A/RConn1 -- Three-Phase V-I Measurement/LConn1

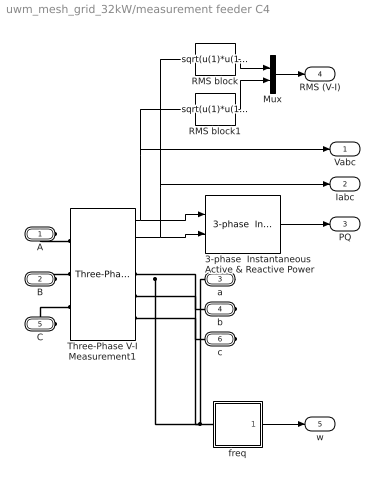
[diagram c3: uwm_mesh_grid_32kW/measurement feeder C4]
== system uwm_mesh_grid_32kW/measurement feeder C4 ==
  3-phase  Instantaneous  Active & Reactive Power : powerlib_extras/Measurements/3-phase  Instantaneous  Active & Reactive Power  DialogController=POWERSYS.PowerSysDialog  SystemSampleTime=-1
  Mux : Mux  Inputs=2
  RMS block : Fcn  Expr=sqrt(u(1)*u(1)+u(2)*u(2)+u(3)*u(3))/sqrt(3)
  RMS block1 : Fcn  Expr=sqrt(u(1)*u(1)+u(2)*u(2)+u(3)*u(3))/sqrt(3)
  Three-Phase V-I Measurement1 : powerlib/Measurements/Three-Phase V-I Measurement  DialogController=POWERSYS.PowerSysDialog  SystemSampleTime=-1  VoltageMeasurement=phase-to-ground  SetLabelV=off  LabelV=Vabc  Vpu=off  VpuLL=off  CurrentMeasurement=yes  SetLabelI=off  LabelI=Iabc  Ipu=off  Pbase=100e6  Vbase=500e3  OutputType=Complex  PhasorSimulation=off  PSBequivalent=0
  freq : Subsystem  AncestorBlock=|
      | UWM_blocks/frequency
      | measurement
      | (zero-crossings)
  A : PMIOPort  Port=1  Side=Left
  B : PMIOPort  Port=2  Side=Left
  a : PMIOPort  Port=3  Side=Right
  b : PMIOPort  Port=4  Side=Right
  C : PMIOPort  Port=5  Side=Left
  c : PMIOPort  Port=6  Side=Right
  Vabc : Outport  OutDataType=fixdt(1, 16)  OutScaling=2^0
  Iabc : Outport  Port=2  OutDataType=fixdt(1, 16)  OutScaling=2^0
  PQ : Outport  Port=3  OutDataType=fixdt(1, 16)  OutScaling=2^0
  RMS (V-I) : Outport  Port=4  OutDataType=fixdt(1, 16)  OutScaling=2^0
  w : Outport  Port=5  OutDataType=fixdt(1, 16)  OutScaling=2^0
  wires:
  Three-Phase V-I Measurement1/1 -> Vabc/1, RMS block1/1, 3-phase  Instantaneous  Active & Reactive Power/1
  Three-Phase V-I Measurement1/2 -> Iabc/1, RMS block/1, 3-phase  Instantaneous  Active & Reactive Power/2
  Mux/1 -> RMS (V-I)/1
  RMS block/1 -> Mux/1
  RMS block1/1 -> Mux/2
  3-phase  Instantaneous  Active & Reactive Power/1 -> PQ/1
  freq/1(w (Hz)) -> w/1
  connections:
  c/RConn1 -- Three-Phase V-I Measurement1/RConn3
  C/RConn1 -- Three-Phase V-I Measurement1/LConn3
  b/RConn1 -- Three-Phase V-I Measurement1/RConn2
  freq/LConn1 -- Three-Phase V-I Measurement1/RConn1 -- a/RConn1
  B/RConn1 -- Three-Phase V-I Measurement1/LConn2
  A/RConn1 -- Three-Phase V-I Measurement1/LConn1

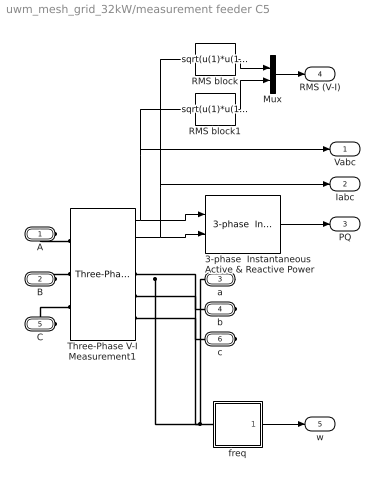
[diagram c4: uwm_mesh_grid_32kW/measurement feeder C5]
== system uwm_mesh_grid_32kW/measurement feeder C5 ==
  3-phase  Instantaneous  Active & Reactive Power : powerlib_extras/Measurements/3-phase  Instantaneous  Active & Reactive Power  DialogController=POWERSYS.PowerSysDialog  SystemSampleTime=-1
  Mux : Mux  Inputs=2
  RMS block : Fcn  Expr=sqrt(u(1)*u(1)+u(2)*u(2)+u(3)*u(3))/sqrt(3)
  RMS block1 : Fcn  Expr=sqrt(u(1)*u(1)+u(2)*u(2)+u(3)*u(3))/sqrt(3)
  Three-Phase V-I Measurement1 : powerlib/Measurements/Three-Phase V-I Measurement  DialogController=POWERSYS.PowerSysDialog  SystemSampleTime=-1  VoltageMeasurement=phase-to-ground  SetLabelV=off  LabelV=Vabc  Vpu=off  VpuLL=off  CurrentMeasurement=yes  SetLabelI=off  LabelI=Iabc  Ipu=off  Pbase=100e6  Vbase=500e3  OutputType=Complex  PhasorSimulation=off  PSBequivalent=0
  freq : Subsystem  AncestorBlock=|
      | UWM_blocks/frequency
      | measurement
      | (zero-crossings)
  A : PMIOPort  Port=1  Side=Left
  B : PMIOPort  Port=2  Side=Left
  a : PMIOPort  Port=3  Side=Right
  b : PMIOPort  Port=4  Side=Right
  C : PMIOPort  Port=5  Side=Left
  c : PMIOPort  Port=6  Side=Right
  Vabc : Outport  OutDataType=fixdt(1, 16)  OutScaling=2^0
  Iabc : Outport  Port=2  OutDataType=fixdt(1, 16)  OutScaling=2^0
  PQ : Outport  Port=3  OutDataType=fixdt(1, 16)  OutScaling=2^0
  RMS (V-I) : Outport  Port=4  OutDataType=fixdt(1, 16)  OutScaling=2^0
  w : Outport  Port=5  OutDataType=fixdt(1, 16)  OutScaling=2^0
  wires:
  Three-Phase V-I Measurement1/1 -> Vabc/1, RMS block1/1, 3-phase  Instantaneous  Active & Reactive Power/1
  Three-Phase V-I Measurement1/2 -> Iabc/1, RMS block/1, 3-phase  Instantaneous  Active & Reactive Power/2
  Mux/1 -> RMS (V-I)/1
  RMS block/1 -> Mux/1
  RMS block1/1 -> Mux/2
  3-phase  Instantaneous  Active & Reactive Power/1 -> PQ/1
  freq/1(w (Hz)) -> w/1
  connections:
  c/RConn1 -- Three-Phase V-I Measurement1/RConn3
  C/RConn1 -- Three-Phase V-I Measurement1/LConn3
  b/RConn1 -- Three-Phase V-I Measurement1/RConn2
  freq/LConn1 -- Three-Phase V-I Measurement1/RConn1 -- a/RConn1
  B/RConn1 -- Three-Phase V-I Measurement1/LConn2
  A/RConn1 -- Three-Phase V-I Measurement1/LConn1

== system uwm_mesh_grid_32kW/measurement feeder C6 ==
  3-phase  Instantaneous  Active & Reactive Power : powerlib_extras/Measurements/3-phase  Instantaneous  Active & Reactive Power  DialogController=POWERSYS.PowerSysDialog  SystemSampleTime=-1
  Mux : Mux  Inputs=2
  RMS block : Fcn  Expr=sqrt(u(1)*u(1)+u(2)*u(2)+u(3)*u(3))/sqrt(3)
  RMS block1 : Fcn  Expr=sqrt(u(1)*u(1)+u(2)*u(2)+u(3)*u(3))/sqrt(3)
  Three-Phase V-I Measurement : powerlib/Measurements/Three-Phase V-I Measurement  DialogController=POWERSYS.PowerSysDialog  SystemSampleTime=-1  VoltageMeasurement=phase-to-ground  SetLabelV=off  LabelV=Vabc  Vpu=off  VpuLL=off  CurrentMeasurement=yes  SetLabelI=off  LabelI=Iabc  Ipu=off  Pbase=100e6  Vbase=500e3  OutputType=Complex  PhasorSimulation=off  PSBequivalent=0
  A : PMIOPort  Port=1  Side=Left
  B : PMIOPort  Port=2  Side=Left
  a : PMIOPort  Port=3  Side=Right
  b : PMIOPort  Port=4  Side=Right
  C : PMIOPort  Port=5  Side=Left
  c : PMIOPort  Port=6  Side=Right
  Vabc : Outport  OutDataType=fixdt(1, 16)  OutScaling=2^0
  Iabc : Outport  Port=2  OutDataType=fixdt(1, 16)  OutScaling=2^0
  PQ : Outport  Port=3  OutDataType=fixdt(1, 16)  OutScaling=2^0
  RMS (V-I) : Outport  Port=4  OutDataType=fixdt(1, 16)  OutScaling=2^0
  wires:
  Three-Phase V-I Measurement/1 -> Vabc/1, RMS block1/1, 3-phase  Instantaneous  Active & Reactive Power/1
  Three-Phase V-I Measurement/2 -> Iabc/1, RMS block/1, 3-phase  Instantaneous  Active & Reactive Power/2
  Mux/1 -> RMS (V-I)/1
  RMS block/1 -> Mux/1
  RMS block1/1 -> Mux/2
  3-phase  Instantaneous  Active & Reactive Power/1 -> PQ/1
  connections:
  c/RConn1 -- Three-Phase V-I Measurement/RConn3
  C/RConn1 -- Three-Phase V-I Measurement/LConn3
  b/RConn1 -- Three-Phase V-I Measurement/RConn2
  a/RConn1 -- Three-Phase V-I Measurement/RConn1
  B/RConn1 -- Three-Phase V-I Measurement/LConn2
  A/RConn1 -- Three-Phase V-I Measurement/LConn1

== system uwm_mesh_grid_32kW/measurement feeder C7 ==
  3-phase  Instantaneous  Active & Reactive Power : powerlib_extras/Measurements/3-phase  Instantaneous  Active & Reactive Power  DialogController=POWERSYS.PowerSysDialog  SystemSampleTime=-1
  Mux : Mux  Inputs=2
  RMS block : Fcn  Expr=sqrt(u(1)*u(1)+u(2)*u(2)+u(3)*u(3))/sqrt(3)
  RMS block1 : Fcn  Expr=sqrt(u(1)*u(1)+u(2)*u(2)+u(3)*u(3))/sqrt(3)
  Three-Phase V-I Measurement : powerlib/Measurements/Three-Phase V-I Measurement  DialogController=POWERSYS.PowerSysDialog  SystemSampleTime=-1  VoltageMeasurement=phase-to-ground  SetLabelV=off  LabelV=Vabc  Vpu=off  VpuLL=off  CurrentMeasurement=yes  SetLabelI=off  LabelI=Iabc  Ipu=off  Pbase=100e6  Vbase=500e3  OutputType=Complex  PhasorSimulation=off  PSBequivalent=0
  A : PMIOPort  Port=1  Side=Left
  B : PMIOPort  Port=2  Side=Left
  a : PMIOPort  Port=3  Side=Right
  b : PMIOPort  Port=4  Side=Right
  C : PMIOPort  Port=5  Side=Left
  c : PMIOPort  Port=6  Side=Right
  Vabc : Outport  OutDataType=fixdt(1, 16)  OutScaling=2^0
  Iabc : Outport  Port=2  OutDataType=fixdt(1, 16)  OutScaling=2^0
  PQ : Outport  Port=3  OutDataType=fixdt(1, 16)  OutScaling=2^0
  RMS (V-I) : Outport  Port=4  OutDataType=fixdt(1, 16)  OutScaling=2^0
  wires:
  Three-Phase V-I Measurement/1 -> Vabc/1, RMS block1/1, 3-phase  Instantaneous  Active & Reactive Power/1
  Three-Phase V-I Measurement/2 -> Iabc/1, RMS block/1, 3-phase  Instantaneous  Active & Reactive Power/2
  Mux/1 -> RMS (V-I)/1
  RMS block/1 -> Mux/1
  RMS block1/1 -> Mux/2
  3-phase  Instantaneous  Active & Reactive Power/1 -> PQ/1
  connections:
  c/RConn1 -- Three-Phase V-I Measurement/RConn3
  C/RConn1 -- Three-Phase V-I Measurement/LConn3
  b/RConn1 -- Three-Phase V-I Measurement/RConn2
  a/RConn1 -- Three-Phase V-I Measurement/RConn1
  B/RConn1 -- Three-Phase V-I Measurement/LConn2
  A/RConn1 -- Three-Phase V-I Measurement/LConn1

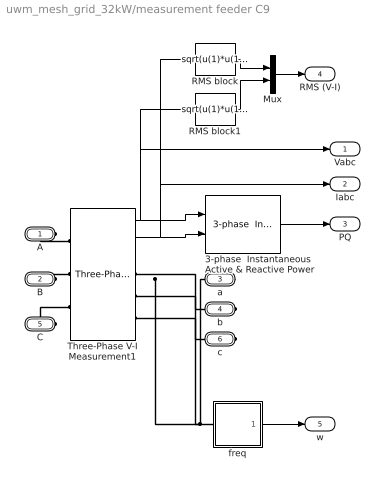
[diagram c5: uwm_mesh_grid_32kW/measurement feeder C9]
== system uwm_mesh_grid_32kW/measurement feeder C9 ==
  3-phase  Instantaneous  Active & Reactive Power : powerlib_extras/Measurements/3-phase  Instantaneous  Active & Reactive Power  DialogController=POWERSYS.PowerSysDialog  SystemSampleTime=-1
  Mux : Mux  Inputs=2
  RMS block : Fcn  Expr=sqrt(u(1)*u(1)+u(2)*u(2)+u(3)*u(3))/sqrt(3)
  RMS block1 : Fcn  Expr=sqrt(u(1)*u(1)+u(2)*u(2)+u(3)*u(3))/sqrt(3)
  Three-Phase V-I Measurement1 : powerlib/Measurements/Three-Phase V-I Measurement  DialogController=POWERSYS.PowerSysDialog  SystemSampleTime=-1  VoltageMeasurement=phase-to-ground  SetLabelV=off  LabelV=Vabc  Vpu=off  VpuLL=off  CurrentMeasurement=yes  SetLabelI=off  LabelI=Iabc  Ipu=off  Pbase=100e6  Vbase=500e3  OutputType=Complex  PhasorSimulation=off  PSBequivalent=0
  freq : Subsystem  AncestorBlock=|
      | UWM_blocks/frequency
      | measurement
      | (zero-crossings)
  A : PMIOPort  Port=1  Side=Left
  B : PMIOPort  Port=2  Side=Left
  a : PMIOPort  Port=3  Side=Right
  b : PMIOPort  Port=4  Side=Right
  C : PMIOPort  Port=5  Side=Left
  c : PMIOPort  Port=6  Side=Right
  Vabc : Outport  OutDataType=fixdt(1, 16)  OutScaling=2^0
  Iabc : Outport  Port=2  OutDataType=fixdt(1, 16)  OutScaling=2^0
  PQ : Outport  Port=3  OutDataType=fixdt(1, 16)  OutScaling=2^0
  RMS (V-I) : Outport  Port=4  OutDataType=fixdt(1, 16)  OutScaling=2^0
  w : Outport  Port=5  OutDataType=fixdt(1, 16)  OutScaling=2^0
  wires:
  Three-Phase V-I Measurement1/1 -> Vabc/1, RMS block1/1, 3-phase  Instantaneous  Active & Reactive Power/1
  Three-Phase V-I Measurement1/2 -> Iabc/1, RMS block/1, 3-phase  Instantaneous  Active & Reactive Power/2
  Mux/1 -> RMS (V-I)/1
  RMS block/1 -> Mux/1
  RMS block1/1 -> Mux/2
  3-phase  Instantaneous  Active & Reactive Power/1 -> PQ/1
  freq/1(w (Hz)) -> w/1
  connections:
  c/RConn1 -- Three-Phase V-I Measurement1/RConn3
  C/RConn1 -- Three-Phase V-I Measurement1/LConn3
  b/RConn1 -- Three-Phase V-I Measurement1/RConn2
  freq/LConn1 -- Three-Phase V-I Measurement1/RConn1 -- a/RConn1
  B/RConn1 -- Three-Phase V-I Measurement1/LConn2
  A/RConn1 -- Three-Phase V-I Measurement1/LConn1

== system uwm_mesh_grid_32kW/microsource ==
  E_req : Inport
  P_req : Inport  Port=2
  10 mH : powerlib/Elements/Three-Phase Series RLC Branch  DialogController=POWERSYS.PowerSysDialog  PhysicalDomain=powersysdomain  SubClassName=unknown  LeftPortType=p1  RightPortType=p1  LConnTagsString=A|B|C  RConnTagsString=A|B|C  BranchType=L  Resistance=.0028  Inductance=5e-3  Capacitance=1e-6  Measurements=None
  Current Measurement : powerlib/Measurements/Current Measurement  DialogController=POWERSYS.PowerSysDialog  SystemSampleTime=-1  PhasorSimulation=off  OutputType=Complex  PSBequivalent=0
  Gain : Gain  Gain=1/(2*pi)  ParameterDataType=fixdt(1, 16)  ParameterScaling=2^0  OutDataType=fixdt(1, 16)  OutScaling=2^0
  Mux : Mux  Inputs=3
  T1 : powerlib/Elements/Three-Phase Transformer (Two Windings)  DialogController=POWERSYS.PowerSysDialog  SystemSampleTime=-1  Winding1Connection=Delta (D1)  UNITS=SI  NominalPower=[ 45e3 , 60 ]  Winding1=[208 0.02688 0.1075/(2*pi*60)]  Winding2Connection=Yg  Winding2=[208 0.005047 .0201/(2*pi*60)]  SetSaturation=off  Rm=100.e6  Lm=7650.8  Saturation=[0 0;1359.8 0.93633;5.6659e+05 1.186]  Hysteresis=off  DataFile='hysteresis'  SetInitialFlux=off  InitialFluxes=[0.62422 -0.62422 0.54618]  Measurements=None  MoreParameters=off  BreakLoop=off  DataType=on  TransfoNumber=1
  Three-Phase V-I Measurement : powerlib/Measurements/Three-Phase V-I Measurement  DialogController=POWERSYS.PowerSysDialog  SystemSampleTime=-1  VoltageMeasurement=phase-to-ground  SetLabelV=off  LabelV=Vabc  Vpu=off  VpuLL=off  CurrentMeasurement=yes  SetLabelI=off  LabelI=Iabc  Ipu=off  Pbase=100e6  Vbase=500e3  OutputType=Complex  PhasorSimulation=off  PSBequivalent=0
  UWM_controller : Subsystem  mask{Vbase=208, Sbase=15000}
  Voltage Measurement : powerlib/Measurements/Voltage Measurement  DialogController=POWERSYS.PowerSysDialog  SystemSampleTime=-1  PhasorSimulation=off  OutputType=Complex  PSBequivalent=0
  microsource : Subsystem
  a : PMIOPort  Port=1  Side=Right
  b : PMIOPort  Port=2  Side=Right
  c : PMIOPort  Port=3  Side=Right
  m : Outport  OutDataType=fixdt(1, 16)  OutScaling=2^0
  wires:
  E_req/1 -> UWM_controller/3(E_req)
  P_req/1 -> UWM_controller/4(P_req)
  Three-Phase V-I Measurement/1 -> UWM_controller/1(v_meas)
  Three-Phase V-I Measurement/2 -> UWM_controller/2(i_meas)
  UWM_controller/1(Vpk) -> microsource/1(Vpk)
  UWM_controller/2(w) -> microsource/2(w), Gain/1
  Mux/1 -> m/1
  Voltage Measurement/1 -> Mux/1
  Current Measurement/1 -> Mux/2
  Gain/1 -> Mux/3
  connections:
  Three-Phase V-I Measurement/RConn2 -- b/RConn1 -- Voltage Measurement/LConn2
  Three-Phase V-I Measurement/RConn3 -- c/RConn1
  Current Measurement/RConn1 -- a/RConn1
  Three-Phase V-I Measurement/RConn1 -- Current Measurement/LConn1 -- Voltage Measurement/LConn1
  10 mH/LConn2 -- microsource/RConn2
  10 mH/LConn1 -- microsource/RConn1
  10 mH/LConn3 -- microsource/RConn3
  T1/LConn1 -- 10 mH/RConn1
  T1/LConn2 -- 10 mH/RConn2
  T1/LConn3 -- 10 mH/RConn3
  T1/RConn1 -- Three-Phase V-I Measurement/LConn1
  T1/RConn2 -- Three-Phase V-I Measurement/LConn2
  T1/RConn3 -- Three-Phase V-I Measurement/LConn3
